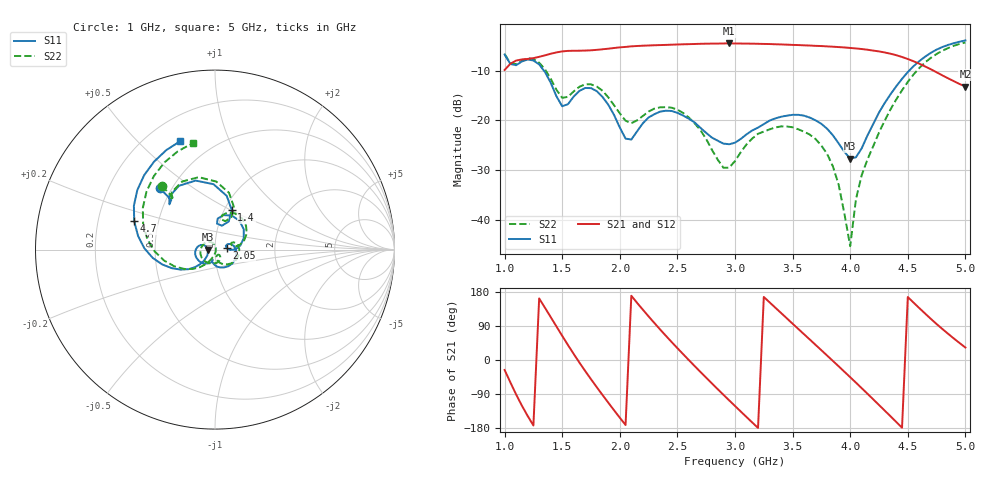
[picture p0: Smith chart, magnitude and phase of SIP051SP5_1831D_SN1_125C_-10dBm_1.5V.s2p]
# GHz  S  dB  R  50
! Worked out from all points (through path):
!   81 points, 1 GHz to 5 GHz, reference 50 ohm
!   highest |S21| = -4.54 dB at 2.95 GHz (marker M1); lowest = -13.2 dB at 5 GHz (marker M2)
!   lowest |S11| = -27.7 dB at 4 GHz (marker M3), VSWR 1.09, Z = 46 + j0.0412 ohm
!   |S11| at or under -10 dB: 1.341 GHz to 4.513 GHz (3.172 GHz wide, 108 % of centre)
!   |S22| runs from -45.3 to -4.4 dB; largest |S21 - S12| = 0.0018
!   S11 on the Smith chart (normalised r, x): 1 GHz: 0.43, +0.37; 1.4 GHz: 1.08, +0.51; 2.05 GHz: 1.14, +0.02; 4.7 GHz: 0.36, +0.15; 5 GHz: 0.33, +0.68
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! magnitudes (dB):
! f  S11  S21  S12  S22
! 1 GHz  -6.8  -9.9  -9.9  -6.7
! 1.1 GHz  -8.9  -8.0  -8.0  -8.7
! 1.25 GHz  -8.0  -7.5  -7.5  -7.7
! 1.4 GHz  -12.4  -6.6  -6.6  -11.6
! 1.5 GHz  -17.2  -6.1  -6.1  -15.5
! 1.7 GHz  -13.5  -6.0  -6.0  -12.8
! 1.85 GHz  -15.3  -5.7  -5.7  -14.1
! 2.05 GHz  -23.7  -5.2  -5.2  -20.1
! 2.35 GHz  -18.2  -4.9  -4.9  -17.4
! 2.6 GHz  -19.7  -4.7  -4.7  -19.5
! 2.95 GHz  -24.8  -4.5  -4.5  -29.5
! 3 GHz  -24.5  -4.6  -4.5  -28.2
! 3.35 GHz  -19.6  -4.7  -4.7  -21.4
! 3.7 GHz  -20.0  -5.0  -5.0  -23.8
! 3.85 GHz  -23.0  -5.2  -5.2  -29.3
! 3.9 GHz  -24.6  -5.3  -5.3  -33.0
! 4 GHz  -27.7  -5.5  -5.5  -45.3
! 4.05 GHz  -27.4  -5.5  -5.6  -35.8
! 4.1 GHz  -25.6  -5.7  -5.7  -31.0
! 4.35 GHz  -14.8  -6.6  -6.6  -17.8
! 4.7 GHz  -6.4  -9.7  -9.7  -7.4
! 5 GHz  -3.9  -13.2  -13.2  -4.4
